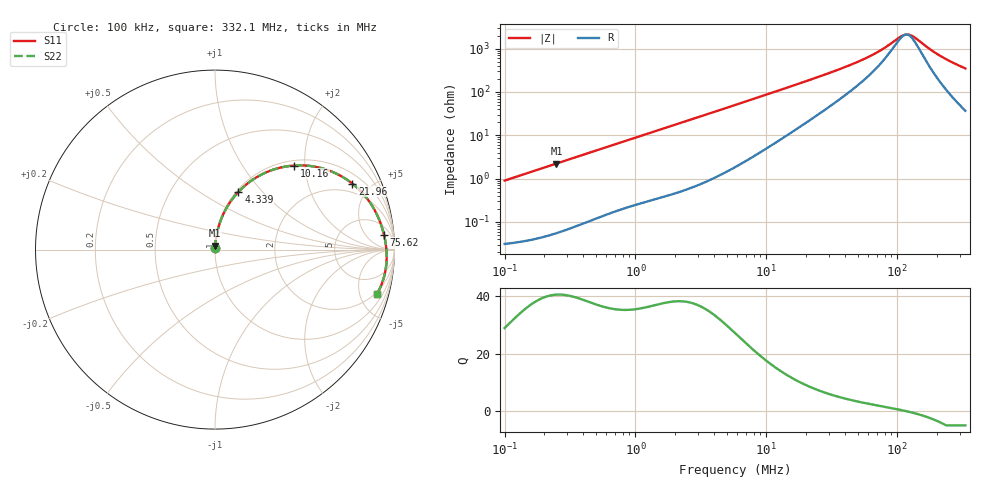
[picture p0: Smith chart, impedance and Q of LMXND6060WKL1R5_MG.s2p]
! LMXND6060WKL1R5_MG  S-PARAMETER MODEL  ( General Type )
! Model Generated by TAIYO YUDEN Corporation (https://www.yuden.co.jp/en/)
! Version 1.0
! TAIYO YUDEN Control No. 191025NI43SB-FBB
! Copyright(c) 2019 TAIYO YUDEN CO.,LTD. All Rights Reserved.
! Product Description (link to TY-COMPAS)
! https://ds.yuden.co.jp/TYCOMPAS/or/detail?pn=LMXND6060WKL1R5NMG&u=M
! Products Name : Inductors
! Characteristics :
!  Inductance : 1.5 uH , SRF(min) : 93 MHz , DC Resistance(max) : 0.0312 Ohm
!  Rated Current : Saturation :4300 mA , Temp Rise : 3600 mA (40 degC)
!  Case Size : 6.0 x 6.0 / 0.236 x 0.236 [mm/inch] , Thickness : 2 / 0.079 [mm/inch]
!  (Conditions: Temperature = 25 degC , DC Bias Current/Voltage = 0A / 0V)
! External Node Assignments :
!  1  o---GGG---o  2
! GND o---------o GND
! Frequency Range : 0.1MHz  -  332.076389MHz  [ 402 STEP ]
# MHz S RI R 50
! Freq[MHz].  S11 Real  S11 Imag  S21 Real  S21 Imag  S12 Real  S12 Imag  S22 Real  S22 Imag
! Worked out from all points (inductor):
!   401 points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, 100 kHz to 332.1 MHz, reference 50 ohm
!   read as one part in series: L = 1.43 uH near 104.1 kHz
!   highest Q = 40.6 at 249 kHz (marker M1), where L = 1.42 uH
!   self-resonance near 116.9 MHz
!   S11 on the Smith chart (normalised r, x): 100 kHz: 1.00, +0.02; 4.339 MHz: 1.02, +0.75; 10.16 MHz: 1.10, +1.76; 21.96 MHz: 1.47, +3.86; 75.62 MHz: 10, +16; 332.1 MHz: 1.74, -6.94
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0.1  0.000391 0.00897  0.9996 -0.00897  0.9996 -0.00897  0.000391 0.00897
0.248966  0.00104 0.0223  0.999 -0.0223  0.999 -0.0223  0.00104 0.0223
0.388873  0.00209 0.0346  0.9979 -0.0346  0.9979 -0.0346  0.00209 0.0346
1.512219  0.0204 0.1284  0.9796 -0.1284  0.9796 -0.1284  0.0204 0.1284
2.722103  0.0579 0.2206  0.9421 -0.2206  0.9421 -0.2206  0.0579 0.2206
4.33886  0.1309 0.3221  0.8691 -0.3221  0.8691 -0.3221  0.1309 0.3221
5.762607  0.2075 0.3876  0.7925 -0.3876  0.7925 -0.3876  0.2075 0.3876
10.16496  0.4408 0.4684  0.5592 -0.4684  0.5592 -0.4684  0.4408 0.4684
14.34691  0.6022 0.4514  0.3978 -0.4514  0.3978 -0.4514  0.6022 0.4514
21.95954  0.7646 0.3682  0.2354 -0.3682  0.2354 -0.3682  0.7646 0.3682
22.4092  0.7708 0.3632  0.2292 -0.3632  0.2292 -0.3632  0.7708 0.3632
30.99387  0.8502 0.2809  0.1498 -0.2809  0.1498 -0.2809  0.8502 0.2809
45.55486  0.9058 0.1876  0.0942 -0.1876  0.0942 -0.1876  0.9058 0.1876
75.61571  0.9416 0.0827  0.0584 -0.0827  0.0584 -0.0827  0.9416 0.0827
87.14324  0.9473 0.0557  0.0527 -0.0557  0.0527 -0.0557  0.9473 0.0557
108.91  0.9536 0.0136  0.0464 -0.0136  0.0464 -0.0136  0.9536 0.0136
118.1082  0.9551 -0.00199  0.0449 0.00199  0.0449 0.00199  0.9551 -0.00199
125.5132  0.9559 -0.0139  0.0441 0.0139  0.0441 0.0139  0.9559 -0.0139
136.1137  0.9565 -0.0301  0.0435 0.0301  0.0435 0.0301  0.9565 -0.0301
177.1504  0.9542 -0.0863  0.0458 0.0863  0.0458 0.0863  0.9542 -0.0863
212.6033  0.9474 -0.1293  0.0526 0.1293  0.0526 0.1293  0.9474 -0.1293
332.0764  0.9018 -0.2493  0.0982 0.2493  0.0982 0.2493  0.9018 -0.2493
